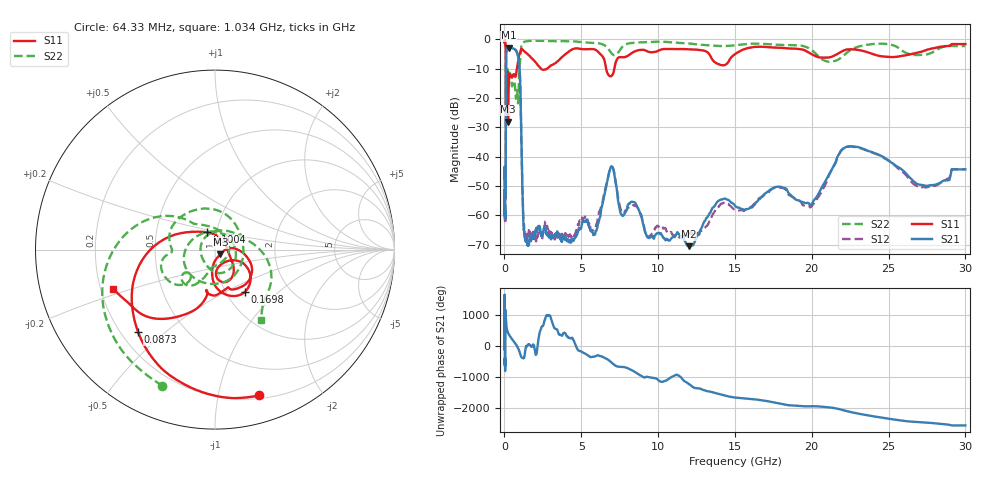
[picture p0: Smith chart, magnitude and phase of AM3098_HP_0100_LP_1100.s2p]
! Date/Time: Thu, Feb 28, 2019 8:35 AM
! Network Analyzer: Agilent Technologies E8364B Rev: A.07.50.67
! Sweep from 0.010 to 30.000 GHz, 1601 Points, Sweep Type: LOG
! Power Supply: 5.023 V, 0.002 A
# Hz S DB R 50
!freq MagS11 AngS11 MagS21 AngS21 MagS12 AngS12 MagS22 AngS22
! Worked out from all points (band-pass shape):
!   1601 points, 10 MHz to 30 GHz, reference 50 ohm
!   highest |S21| = -2.80 dB at 267.8 MHz (marker M1); lowest = -70.5 dB at 12.01 GHz (marker M2)
!   |S21| within 3 dB of the highest: 112 MHz to 888.3 MHz (776.3 MHz wide, 155 % of centre)
!   lowest |S11| = -28.0 dB at 236.3 MHz (marker M3), VSWR 1.08, Z = 53.1 - j2.7 ohm
!   |S11| at or under -10 dB: 95.97 MHz to 811.8 MHz (715.8 MHz wide, 158 % of centre); 2.373 GHz to 2.771 GHz (398.3 MHz wide, 15.5 % of centre); 6.616 GHz to 7.153 GHz (536.9 MHz wide, 7.8 % of centre)
!   |S22| runs from -22.4 to -0.5 dB; largest |S21 - S12| = 0.011
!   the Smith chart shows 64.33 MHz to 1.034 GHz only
!   S11 on the Smith chart (normalised r, x): 64.33 MHz: 0.23, -1.32; 87.3 MHz: 0.27, -0.41; 100.4 MHz: 0.90, +0.18; 169.8 MHz: 1.23, -0.63; 1.034 GHz: 0.25, -0.18
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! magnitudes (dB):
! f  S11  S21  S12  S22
! 10 MHz  -0.4  -47.5  -43.2  -0.6
! 38.04 MHz  -0.5  -60.0  -59.5  -1.0
! 64.33 MHz  -1.4  -52.5  -53.5  -1.8
! 76.65 MHz  -2.1  -51.9  -53.1  -2.6
! 87.3 MHz  -4.0  -35.0  -34.8  -4.5
! 100.4 MHz  -19.4  -11.1  -11.1  -21.7
! 144.7 MHz  -16.9  -3.6  -3.6  -13.5
! 169.8 MHz  -10.8  -3.4  -3.4  -10.2
! 236.3 MHz  -28.0  -2.9  -2.9  -12.2
! 267.8 MHz  -17.5  -2.8  -2.8  -12.4
! 550.5 MHz  -12.3  -3.1  -3.0  -14.9
! 885.5 MHz  -7.8  -5.7  -5.7  -21.7
! 1.034 GHz  -4.3  -16.7  -16.7  -6.5
! 1.276 GHz  -4.0  -65.5  -63.7  -0.9
! 2.084 GHz  -8.2  -64.6  -67.5  -0.5
! 5.812 GHz  -3.3  -66.7  -65.0  -1.2
! 6.924 GHz  -12.6  -43.5  -43.5  -4.4
! 7.926 GHz  -5.9  -58.5  -58.1  -1.6
! 12.01 GHz  -3.4  -70.5  -66.4  -1.4
! 19.9 GHz  -4.7  -56.4  -57.3  -3.3
! 22.56 GHz  -3.4  -36.4  -36.6  -3.5
! 30 GHz  -1.6  -44.3  -44.3  -2.3
